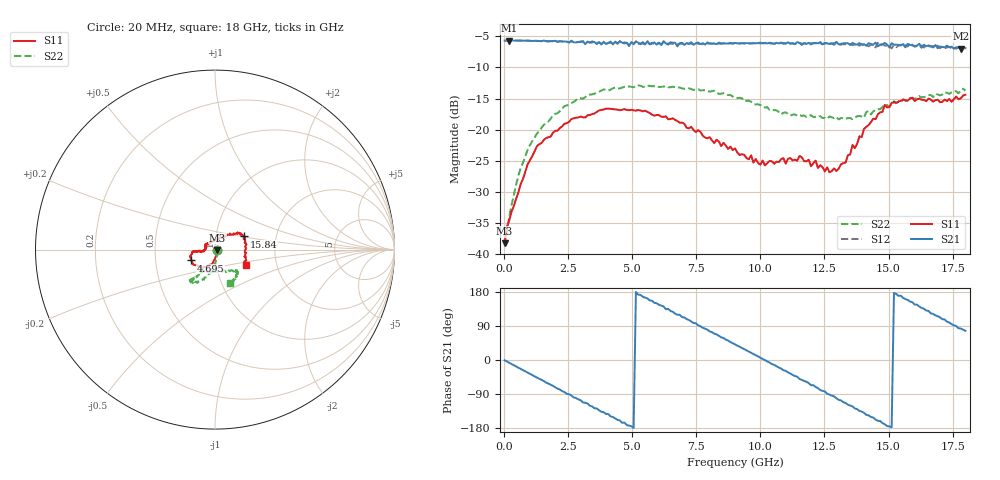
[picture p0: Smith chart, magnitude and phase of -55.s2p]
!Agilent Technologies,N5230A,US43500223,A.07.50.48
!Agilent N5230A: A.07.50.48
!Date: Sunday, January 31, 2016 13:37:55
!Correction: S11(Full 2 Port(1,2))
!S21(Full 2 Port(1,2))
!S12(Full 2 Port(1,2))
!S22(Full 2 Port(1,2))
!S2P File: Measurements: S11, S21, S12, S22:
# Hz S  dB  R 50
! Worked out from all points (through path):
!   201 points, 20 MHz to 18 GHz, reference 50 ohm
!   highest |S21| = -5.68 dB at 199.8 MHz (marker M1); lowest = -7.0 dB at 17.82 GHz (marker M2)
!   group delay of S21, straight-line fit = 99.1 ps
!   lowest |S11| = -38.2 dB at 20 MHz (marker M3), VSWR 1.02, Z = 51.2 - j0.254 ohm
!   |S11| at or under -10 dB: start of sweep to end of sweep
!   |S22| runs from -38.7 to -12.9 dB; largest |S21 - S12| = 0.059
!   S11 on the Smith chart (normalised r, x): 20 MHz: 1.02, -0.01; 4.695 GHz: 0.76, -0.09; 15.84 GHz: 1.37, +0.21; 18 GHz: 1.39, -0.25
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2e7  -38.22 -11.6  -5.68 -0.7  -5.69 -0.9  -38.70 -12.7
1.998e8  -34.56 -39.4  -5.68 -7.2  -5.67 -7.3  -34.04 -51.3
6.493e8  -28.70 -80.1  -5.70 -23.6  -5.70 -23.6  -26.15 -80.1
1.1887e9  -23.48 -97.2  -5.72 -43.0  -5.75 -43.2  -21.24 -91.0
1.9978e9  -20.16 -112.6  -5.72 -72.1  -5.76 -72.3  -17.45 -102.3
3.0766e9  -18.01 -130.4  -5.77 -112.2  -5.87 -111.4  -15.01 -112.4
4.6948e9  -16.70 -155.7  -6.14 -165.2  -5.96 -167.1  -13.11 -124.1
5.5938e9  -17.13 -165.8  -5.78 162.3  -6.07 160.3  -12.95 -127.9
6.0433e9  -17.65 -171.6  -6.00 145.6  -6.13 143.2  -13.14 -128.0
7.5716e9  -20.07 -173.0  -5.98 91.4  -6.21 90.4  -13.51 -128.2
9.01e9  -23.00 -174.1  -6.06 41.4  -6.12 39.3  -14.84 -124.7
9.7292e9  -25.28 -179.8  -6.11 15.7  -6.12 13.7  -15.87 -122.6
1.06282e10  -25.13 167.0  -6.04 -16.4  -6.11 -18.6  -16.89 -118.9
1.20666e10  -25.38 141.5  -6.13 -66.5  -6.06 -71.1  -17.98 -107.3
1.29656e10  -26.64 102.2  -5.87 -100.8  -6.14 -105.5  -17.95 -95.7
1.37747e10  -22.27 58.6  -6.34 -129.6  -6.14 -134.8  -17.84 -74.0
1.44939e10  -18.31 43.5  -6.00 -157.3  -6.78 -158.1  -16.82 -56.3
1.50333e10  -16.39 35.1  -6.79 -175.2  -6.60 179.1  -16.33 -46.3
1.58424e10  -14.98 24.4  -6.39 154.2  -6.16 152.4  -14.92 -44.9
1.69212e10  -15.18 2.8  -6.91 115.2  -6.50 110.5  -14.32 -54.7
1.78202e10  -14.95 -23.8  -6.99 82.9  -7.09 77.2  -13.67 -60.4
1.8e10  -14.39 -26.5  -6.89 76.9  -6.97 70.6  -13.74 -66.1
